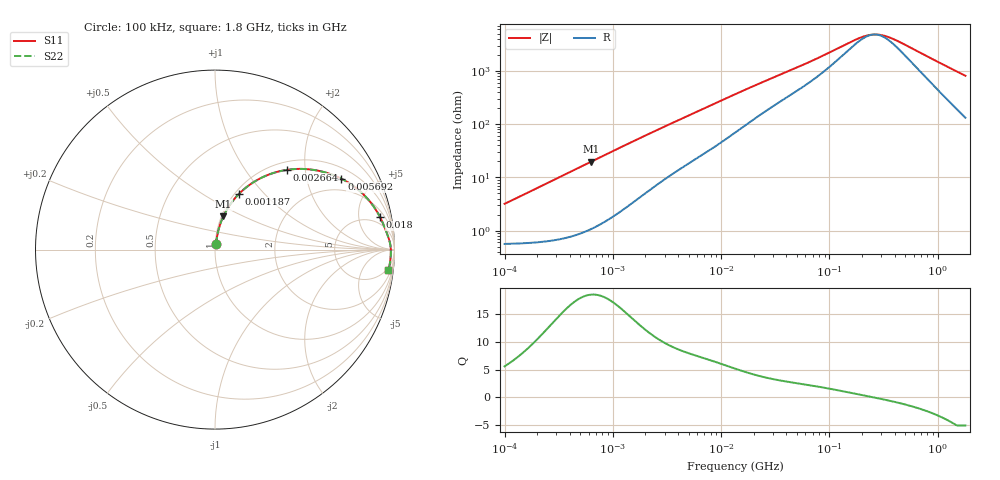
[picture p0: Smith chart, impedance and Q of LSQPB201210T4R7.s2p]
! LSQPB201210T4R7  S-PARAMETER MODEL  ( General Type )
! Model Generated by TAIYO YUDEN Corporation (http://www.ty-top.com)
! Version 2.0
! TAIYO YUDEN Control No. 100810NF18SB-HKC
! Copyright(c) 2007 TAIYO YUDEN CO.,LTD. All Rights Reserved.
! Product Description (link to TY-COMPAS)
! https://ds.yuden.co.jp/TYCOMPAS/or/detail?pn=LSQPB201210T4R7M&u=M
! Products Name : Inductors
! Characteristics :
!  Inductance : 4.7 uH , SRF(min) : 150 MHz , DC Resistance(max) : 0.715 Ohm
!  Rated Current : Saturation :340 mA , Temp Rise : 400 mA (40 degC)
!  Case Size : 2.0 x 1.25 / 0.079 x 0.049 [mm/inch] , Thickness : 1.0 / 0.04 [mm/inch]
!  (Conditions: Temperature = 25 degC , DC Bias Current/Voltage = 0A / 0V)
! External Node Assignments :
!  1  o---GGG---o  2
! GND o---------o GND
! Frequency Range : 0.1MHz  -  1800MHz  [ 402 STEP ]
# MHz S RI R 50
! Freq[MHz].  S11 Real  S11 Imag  S21 Real  S21 Imag  S12 Real  S12 Imag  S22 Real  S22 Imag
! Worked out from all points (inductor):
!   401 points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, 100 kHz to 1.8 GHz, reference 50 ohm
!   read as one part in series: L = 5 uH near 105 kHz
!   highest Q = 18.4 at 627.9 kHz (marker M1), where L = 4.98 uH
!   self-resonance near 259.1 MHz
!   S11 on the Smith chart (normalised r, x): 100 kHz: 1.01, +0.06; 1.187 MHz: 1.05, +0.74; 2.664 MHz: 1.15, +1.60; 5.692 MHz: 1.43, +3.25; 18 MHz: 3.12, +9.27; 1.8 GHz: 4, -16
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0.1  0.00657 0.031  0.9934 -0.031  0.9934 -0.031  0.00657 0.031
0.247521  0.0122 0.0763  0.9878 -0.0763  0.9878 -0.0763  0.0122 0.0763
0.516129  0.0338 0.1549  0.9662 -0.1549  0.9662 -0.1549  0.0338 0.1549
0.627861  0.0466 0.1854  0.9534 -0.1854  0.9534 -0.1854  0.0466 0.1854
0.884704  0.0832 0.2493  0.9168 -0.2493  0.9168 -0.2493  0.0832 0.2493
1.187015  0.135 0.3118  0.865 -0.3118  0.865 -0.3118  0.135 0.3118
1.714072  0.235 0.3878  0.765 -0.3878  0.765 -0.3878  0.235 0.3878
2.66389  0.4028 0.4446  0.5972 -0.4446  0.5972 -0.4446  0.4028 0.4446
3.846706  0.5576 0.4428  0.4424 -0.4428  0.4424 -0.4428  0.5576 0.4428
5.692459  0.7047 0.3948  0.2953 -0.3948  0.2953 -0.3948  0.7047 0.3948
8.632747  0.8192 0.3149  0.1808 -0.3149  0.1808 -0.3149  0.8192 0.3149
13.41641  0.8918 0.2287  0.1082 -0.2287  0.1082 -0.2287  0.8918 0.2287
18.00091  0.9199 0.1802  0.0801 -0.1802  0.0801 -0.1802  0.9199 0.1802
32.40491  0.9507 0.11  0.0493 -0.11  0.0493 -0.11  0.9507 0.11
69.24595  0.9702 0.055  0.0298 -0.055  0.0298 -0.055  0.9702 0.055
167.2511  0.9786 0.0153  0.0214 -0.0153  0.0214 -0.0153  0.9786 0.0153
213.6735  0.9794 0.0066  0.0206 -0.0066  0.0206 -0.0066  0.9794 0.0066
272.9811  0.9798 -0.00179  0.0202 0.00179  0.0202 0.00179  0.9798 -0.00179
357.3983  0.9799 -0.0112  0.0201 0.0112  0.0201 0.0112  0.9799 -0.0112
456.5984  0.9797 -0.0205  0.0203 0.0205  0.0203 0.0205  0.9797 -0.0205
884.6373  0.9774 -0.0535  0.0226 0.0535  0.0226 0.0535  0.9774 -0.0535
1800  0.9665 -0.1154  0.0335 0.1154  0.0335 0.1154  0.9665 -0.1154
